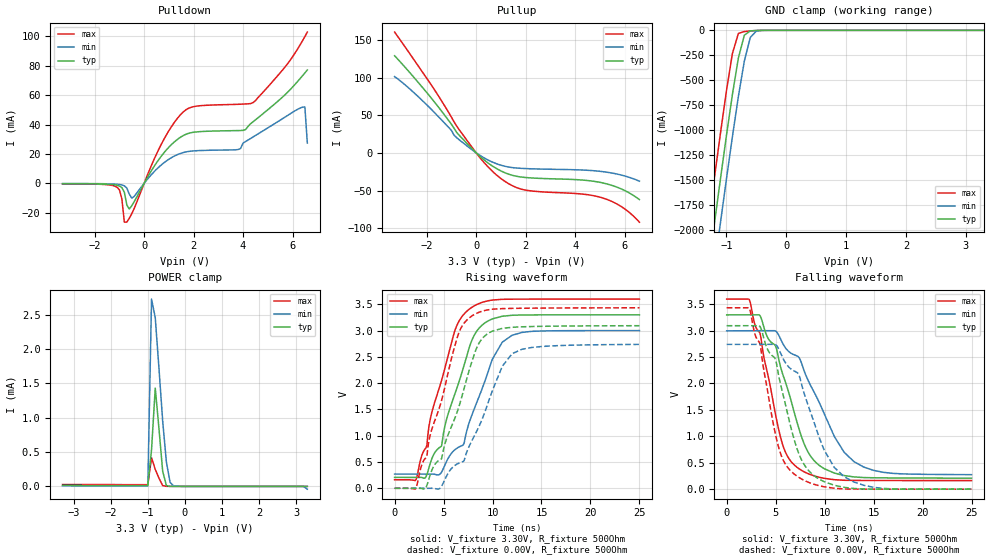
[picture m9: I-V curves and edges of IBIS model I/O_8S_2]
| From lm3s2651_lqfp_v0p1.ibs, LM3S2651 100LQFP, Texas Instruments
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[Model]   I/O_8S_2
Model_type   I/O
Vinl = 1.26
Vinh = 2.04
Vmeas = 1.65
| variable   typ   min   max
C_comp   9.739pF   9.739pF   9.739pF
[Model Spec]
Vinh+   1.91   1.78   2.04
Vinh-   1.90   1.76   2.03
Vinl+   1.40   1.27   1.54
Vinl-   1.39   1.26   1.53
| variable   typ   min   max
[Temperature Range]  25   85   -40
[Voltage Range]   3.3V   3.0V   3.6V
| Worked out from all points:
|   slope of the pulldown table from 0 to 0.495 V, typ, clamps not added: 35.8 ohm
|   slope of the pullup table from 0 to 0.495 V, typ, clamps not added: 35.8 ohm
|   GND clamp passes 1 mA (typ) near -0.48 V on its own axis
|   POWER clamp passes 1 mA (typ) near -0.73 V on its own axis
|   falling waveform, V_fixture 3.30V, R_fixture 500Ohm: 20-80 % time 2.94ns typ, 4.09ns min, 2.26ns max; typ from 3.3 V to 0.208 V
|   rising waveform, V_fixture 3.30V, R_fixture 500Ohm: 20-80 % time 2.82ns typ, 3.05ns min, 2.7ns max; typ from 0.208 V to 3.3 V
|   falling waveform, V_fixture 0.00V, R_fixture 500Ohm: 20-80 % time 2.56ns typ, 3.29ns min, 2.08ns max; typ from 3.09 V to 0 V
|   rising waveform, V_fixture 0.00V, R_fixture 500Ohm: 20-80 % time 3.14ns typ, 3.58ns min, 2.87ns max; typ from 0 V to 3.09 V
[Pulldown]
|  Voltage   I(typ)   I(min)   I(max)
-3.3V     -256.6uA   -145.6uA   -364.5uA
-1.1V     -1.273mA   -587.5uA   -2.567mA
-900mV    -2.885mA   -1.061mA   -10.54mA
-800mV    -5.993mA   -1.67mA    -26.39mA
-700mV    -14.71mA   -3.215mA   -26.33mA
-500mV    -15.26mA   -10mA      -20.66mA
600mV     16.36mA    11.13mA    23.41mA
1.5V      31.68mA    20.52mA    47.2mA
3.8V      35.88mA    22.99mA    53.74mA
4.4V      41.81mA    31.48mA    54.89mA
6.5V      75.06mA    51.95mA    99.78mA
6.6V      77.08mA    27.42mA    102.8mA
[Pullup]
|  Voltage   I(typ)   I(min)   I(max)
-3.3V     128.9mA    101.3mA    160.4mA
-2V       80.13mA    63.77mA    99.04mA
-1V       37.9mA     29.83mA    47.32mA
-700mV    23.81mA    17.7mA     31.28mA
300mV     -8.845mA   -6.303mA   -12.15mA
1V        -23.99mA   -16.37mA   -34.1mA
1.5V      -30.13mA   -19.7mA    -44.22mA
2V        -32.73mA   -20.87mA   -49.46mA
4.3V      -36.12mA   -22.8mA    -54.75mA
5.1V      -39.81mA   -24.88mA   -59.77mA
5.9V      -48.4mA    -29.75mA   -72.06mA
6.6V      -62.06mA   -37.61mA   -92.08mA
[GND Clamp]
|  Voltage   I(typ)   I(min)   I(max)
-3.3V     -11.72A    -12.12A    -11.3A
-1.4V     -2.845A    -3.285A    -2.387A
-1.3V     -2.39A     -2.831A    -1.93A
-1.2V     -1.938A    -2.38A     -1.478A
-1.1V     -1.494A    -1.934A    -1.036A
-1V       -1.059A    -1.496A    -610.6mA
-900mV    -645mA     -1.069A    -232.9mA
-800mV    -277.1mA   -664.4mA   -31.59mA
-700mV    -48.56mA   -306.6mA   -12.09mA
-600mV    -5.558mA   -70.2mA    -6.272mA
-500mV    -1.167mA   -7.88mA    -2.167mA
3.3V      2.282nA    3.101uA    451.3pA
[POWER Clamp]
|  Voltage   I(typ)   I(min)   I(max)
-3.3V     15.18uA    8.315uA    27.48uA
-1V       14.14uA    7.74uA     25.63uA
-900mV    536uA      2.726mA    416.7uA
-800mV    1.43mA     2.454mA    247.6uA
-700mV    840.7uA    1.719mA    119.9uA
-600mV    221.2uA    951.5uA    11.58uA
-500mV    12.35uA    355.6uA    955.3nA
-400mV    305.2nA    58.59uA    44.3nA
-300mV    9.515nA    3.101uA    1.472nA
3.1V      1.302nA    -112.7nA   143.5pA
3.2V      1.207nA    -2.287uA   131.7pA
3.3V      -104.8pA   -40.34uA   119.2pA
[Ramp]
| variable   typ   min   max
dV/dt_f   1.85/2.94n   1.63/4.09n   2.06/2.26n
dV/dt_r   1.85/3.14n   1.64/3.58n   2.06/2.87n
R_load = 500Ohm
[Falling Waveform]
V_fixture = 3.30V
V_fixture_min = 3.00V
V_fixture_max = 3.60V
R_fixture = 500Ohm
|   Time   V(typ)   V(min)   V(max)
0s        3.298V     2.996V     3.597V
2.3ns     3.298V     2.998V     3.592V
3.4ns     3.285V     2.998V     2.951V
5ns       2.706V     2.991V     1.401V
5.6ns     2.248V     2.805V     914.8mV
7.3ns     1.193V     2.509V     397.4mV
9.2ns     490.2mV    1.738V     237.3mV
11ns      304.1mV    994.2mV    179.2mV
13ns      231.5mV    521mV      165.4mV
25ns      208.4mV    274.1mV    162.4mV
[Rising Waveform]
V_fixture = 3.30V
V_fixture_min = 3.00V
V_fixture_max = 3.60V
R_fixture = 500Ohm
|   Time   V(typ)   V(min)   V(max)
0s        207.7mV    271.2mV    162.2mV
2.1ns     207.6mV    270.5mV    145.4mV
3.2ns     219.5mV    270.2mV    767.1mV
4.8ns     809.5mV    310.2mV    2.056V
6.1ns     1.764V     724.7mV    2.965V
7ns       2.281V     823mV      3.293V
7.7ns     2.72V      1.294V     3.417V
10ns      3.222V     2.461V     3.58V
12ns      3.29V      2.91V      3.596V
25ns      3.299V     2.999V     3.598V
[Falling Waveform]
V_fixture = 0.00V
V_fixture_min = 0.00V
V_fixture_max = 0.00V
R_fixture = 500Ohm
|   Time   V(typ)   V(min)   V(max)
0s        3.093V     2.739V     3.433V
2.3ns     3.093V     2.74V      3.428V
3.4ns     3.081V     2.74V      2.75V
5.3ns     2.158V     2.657V     795.1mV
7.1ns     811.9mV    2.216V     256.2mV
8.2ns     389.8mV    1.652V     141.9mV
10ns      137.8mV    724.8mV    43.49mV
12ns      34.21mV    235.5mV    4mV
16ns      400.8uV    14.31mV    285uV
25ns      39.28uV    92.37uV    23.51uV
[Rising Waveform]
V_fixture = 0.00V
V_fixture_min = 0.00V
V_fixture_max = 0.00V
R_fixture = 500Ohm
|   Time   V(typ)   V(min)   V(max)
0s        386.9uV    2.264mV    176uV
2.1ns     185.3uV    936.1uV    -16.2mV
3.2ns     13.7mV     510.3uV    580.9mV
4.6ns     539.8mV    -3.563mV   1.547V
6.4ns     1.457V     463.1mV    2.869V
7.8ns     2.356V     871.9mV    3.265V
9.2ns     2.896V     1.442V     3.381V
11ns      3.041V     2.321V     3.417V
12ns      3.062V     2.56V      3.421V
25ns      3.092V     2.736V     3.432V
